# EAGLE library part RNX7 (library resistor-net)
RESISTOR NETWORK
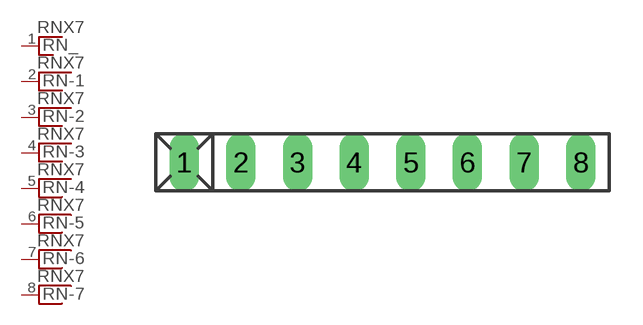
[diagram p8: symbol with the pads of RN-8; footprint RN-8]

Designator prefix RN; gates _=RN_1 -1=RNX -2=RNX -3=RNX -4=RNX -5=RNX -6=RNX -7=RNX

## RNX7 (OC_FARNELL: unknown; OC_NEWARK: unknown)  [RN-8]
1  _:1  pas
2  -1:1  pas
3  -2:1  pas
4  -3:1  pas
5  -4:1  pas
6  -5:1  pas
7  -6:1  pas
8  -7:1  pas

## Footprint RN-8 (pad centres in mm)
RESISTOR NETWORK
drill 0.813 long: 1 -8.89,0; 2 -6.35,0; 3 -3.81,0; 4 -1.27,0; 5 1.27,0; 6 3.81,0; 7 6.35,0; 8 8.89,0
